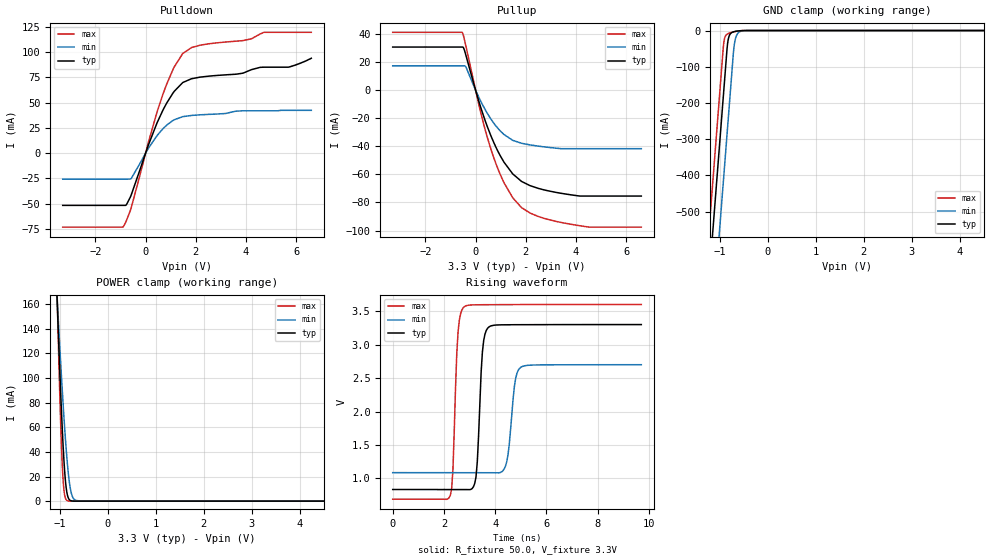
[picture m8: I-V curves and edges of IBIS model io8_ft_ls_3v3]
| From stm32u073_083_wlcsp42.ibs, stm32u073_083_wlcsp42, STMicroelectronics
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[Model]   io8_ft_ls_3v3
Model_type I/O
Polarity   Non-Inverting
Enable   Active-Low
| CAP_THRESHOLD on pad IOFT is "UDTCAPC" :
| Rising=30.0% of vddiom   Falling=70.0% of vddiom
| C_comp min and max val. don't necessarily correlate with the min and max pvt
| but are the smallest and greatest pad capacitance found.
| var   typ   min   max
C_comp   2.27871pF  2.22734pF  2.30488pF
|C_comp_pullup   1.28451pF  1.24023pF  1.22997pF
|C_comp_pulldown   994.19846fF  987.10749fF  1.07492pF
Vinl = 810.0mV
Vinh = 2.52V
Vmeas = 1.65V   | Reference voltage for timing measurements
Cref  = 50.0pF   | Timing specification test load capacitance value
Rref  = 100.0MOhm   | Timing specification test load resistance value
Vref  = 1.65V   | Timing specification test load voltage
[Model Spec]
| TIME_THRESHOLD on pin ZIV12 is "CMOS" :
| Rising=50.0% of vdd   Falling=50.0% of vdd
Vinl 1.34770V 1.11370V 1.44970V
Vinh 1.77530V 1.49030V 1.90330V
| variable   typ   min   max
[Temperature Range] 25.0 125.0 -40.0
| variable   typ   min   max
[Voltage Range] 3.3V 2.7V 3.6V
| variable   typ   min   max
[POWER Clamp Reference] 3.3V 2.7V 3.6V
| variable   typ   min   max
[GND Clamp Reference] 0V 0V 0V
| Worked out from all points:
|   slope of the pulldown table from 0 to 0.495 V, typ, clamps not added: 15.4 ohm
|   slope of the pullup table from 0 to 0.495 V, typ, clamps not added: 18.2 ohm
|   GND clamp passes 1 mA (typ) near -0.60 V on its own axis
|   POWER clamp passes 1 mA (typ) near -0.80 V on its own axis
|   rising waveform, R_fixture 50.0, V_fixture 3.3V: 20-80 % time 176ps typ, 233ps min, 161ps max; typ from 0.835 V to 3.3 V
[POWER Clamp]
-3.3V     3.015A     2.054A     3.978A
-1.06V    166.8mA    167.3mA    172.4mA
-1.05V    156mA      159.9mA    156.7mA
-980mV    85.12mA    110.1mA    59.21mA
-940mV    50.68mA    83.63mA    21.78mA
-920mV    36.19mA    71.13mA    10.91mA
-890mV    19.13mA    53.62mA    3.147mA
-840mV    4.466mA    28.96mA    309.8uA
-790mV    763.7uA    12.17mA    28.67uA
-740mV    119.7uA    3.892mA    2.636uA
-560mV    142.6nA    28.01uA    517.5pA
6.6V      0A         0A         0A
[GND Clamp]
-3.3V     -4.214A    -4.451A    -4.077A
-1.25V    -729.3mA   -965.7mA   -592.4mA
-930mV    -185.3mA   -421.7mA   -48.36mA
-910mV    -151.3mA   -387.7mA   -26.77mA
-890mV    -117.3mA   -353.7mA   -16.93mA
-850mV    -49.27mA   -285.7mA   -10.06mA
-820mV    -21.33mA   -234.7mA   -8.08mA
-720mV    -3.801mA   -64.65mA   -4.026mA
-700mV    -3.065mA   -39.82mA   -3.372mA
-650mV    -1.789mA   -12.81mA   -1.967mA
-550mV    -403.6uA   -1.595mA   -350.4uA
6.6V      834.1pA    91.02nA    597.5pA
| variable   typ   min   max
[Pullup Reference] 3.3V 2.7V 3.6V
| variable   typ   min   max
[Pulldown Reference] 0V 0V 0V
[Pullup]
-3.3V     30.64mA    17.23mA    41.13mA
-530mV    30.64mA    17.23mA    41.01mA
-470mV    29.67mA    17.23mA    37.87mA
-380mV    24.45mA    16.13mA    30.84mA
210mV     -12.56mA   -8.05mA    -16.33mA
640mV     -33.81mA   -21.37mA   -43.64mA
1.14V     -51.54mA   -31.73mA   -66.22mA
1.48V     -59.67mA   -35.78mA   -76.65mA
1.83V     -65.01mA   -37.85mA   -83.65mA
2.51V     -70.03mA   -39.93mA   -90.06mA
3.88V     -74.77mA   -41.71mA   -95.78mA
6.6V      -75.43mA   -41.71mA   -97.57mA
[Pulldown]
-3.3V     -51.64mA   -25.66mA   -73.18mA
-880mV    -51.64mA   -25.66mA   -72.45mA
-570mV    -41.2mA    -25.04mA   -53.78mA
120mV     8.582mA    5.119mA    11.54mA
690mV     42.49mA    24.14mA    58.21mA
1.09V     59.44mA    32.3mA     82.71mA
1.48V     69.88mA    36.14mA    98.63mA
2.17V     75.22mA    37.94mA    106.8mA
3.88V     79.15mA    41.94mA    111.3mA
4.71V     85.07mA    41.94mA    119.6mA
5.7V      85.1mA     42.4mA     119.6mA
6.6V      93.9mA     42.4mA     119.6mA
[Ramp]
dV/dt_r 1.39485V/24.15282ns 945.1373mV/53.90777ns 1.64323V/14.42053ns
dV/dt_f 1.47909V/21.04333ns 967.87468mV/44.44389ns 1.74612V/13.55867ns
R_load = 50.0
| Removed startup time: 0s 0s 0s  .
| Removed end time: 9.75ns.
[Rising Waveform]
R_fixture   = 50.0
V_fixture   = 3.3V
V_fixture_min = 2.7V
V_fixture_max = 3.6V
0s        834.9mV    1.087V     689.8mV
2.25ns    834.9mV    1.087V     751.9mV
2.55ns    834.9mV    1.087V     3.19V
2.8ns     834.3mV    1.087V     3.567V
3.25ns    1.022V     1.087V     3.595V
3.5ns     2.891V     1.087V     3.596V
3.75ns    3.262V     1.086V     3.596V
4.4ns     3.296V     1.185V     3.597V
5ns       3.297V     2.661V     3.598V
9.7ns     3.299V     2.7V       3.599V
